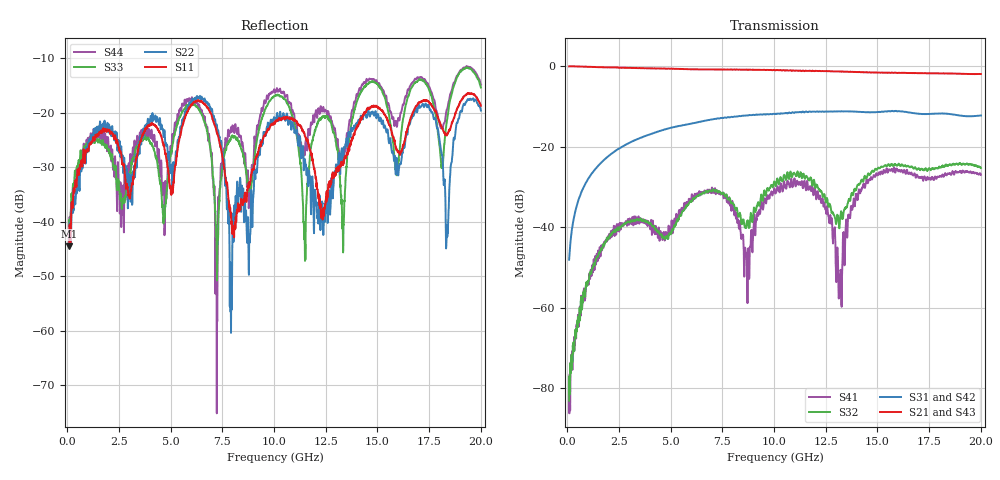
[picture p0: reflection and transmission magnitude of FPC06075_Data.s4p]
! 1/29/2015 6:15:05 AM
! D:\6075\1.S4P
! CHANNEL.1
! TR.MEASUREMENT
! CORRECTED.DATA
# GHZ S RI R 50.0
! FREQ.GHZ  S11RE  S11IM  S12RE  S12IM  S13RE  S13IM  S14RE  S14IM
!  S21RE  S21IM  S22RE  S22IM  S23RE  S23IM  S24RE  S24IM
!  S31RE  S31IM  S32RE  S32IM  S33RE  S33IM  S34RE  S34IM
!  S41RE  S41IM  S42RE  S42IM  S43RE  S43IM  S44RE  S44IM
!; PortSelection: Port_1234
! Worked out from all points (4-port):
!   2000 points, 100 MHz to 20 GHz, reference 50 ohm
!   strongest paths, dB at 100 MHz, 5.077 GHz, 10.05 GHz, 15.03 GHz, 20 GHz:
!     S21: 0.0, -0.6, -1.0, -1.6, -1.9
!     S43: 0.0, -0.7, -1.3, -1.8, -2.1
!     S31: -48.0, -15.2, -11.9, -11.4, -12.2
!     S42: -47.9, -15.2, -12.2, -11.3, -12.1
!     S32: -83.0, -40.5, -29.1, -25.2, -25.2
!     S41: -81.3, -39.7, -31.4, -26.9, -27.0
!   lowest |S11| = -44.5 dB at 100 MHz (marker M1), VSWR 1.01, Z = 49.9 + j0.591 ohm
!   |S11| at or under -10 dB: start of sweep to end of sweep
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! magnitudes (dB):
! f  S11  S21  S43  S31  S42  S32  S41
! 100 MHz  -44.5  0.0  0.0  -48.0  -47.9  -83.0  -81.3
! 2.748 GHz  -29.5  -0.4  -0.4  -19.8  -19.7  -39.3  -39.1
! 7.945 GHz  -40.4  -0.8  -1.0  -12.6  -12.7  -33.9  -35.9
! 10.15 GHz  -21.4  -0.9  -1.3  -11.8  -12.3  -27.9  -30.0
! 11.4 GHz  -23.3  -1.1  -1.3  -11.3  -11.3  -26.7  -30.2
! 13.2 GHz  -29.7  -1.3  -1.5  -11.2  -11.1  -37.6  -52.7
! 20 GHz  -18.7  -1.9  -2.1  -12.2  -12.1  -25.2  -27.0
